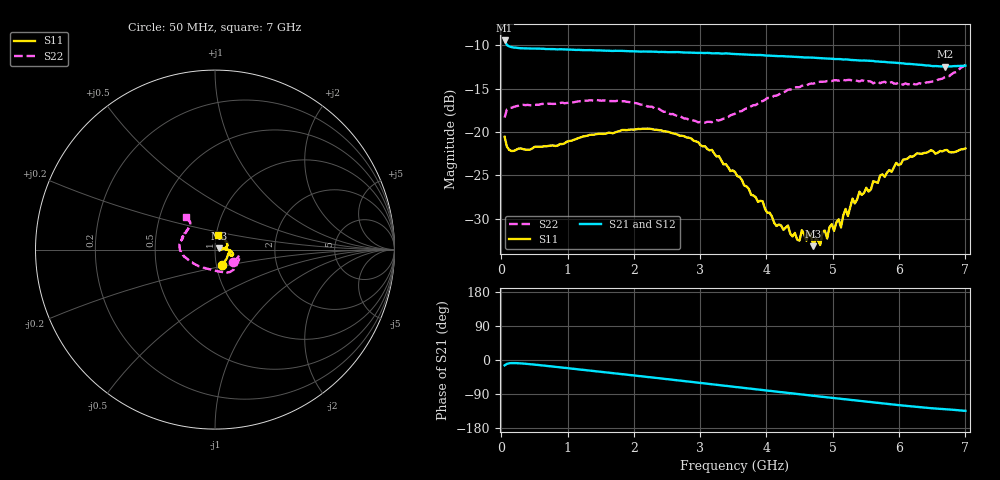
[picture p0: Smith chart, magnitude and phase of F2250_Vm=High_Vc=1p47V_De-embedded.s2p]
! Integrated Device Technology
! Corporate Headquarters
! 6024 Silver Creek Valley Road
! San Jose, CA 95138  USA
! Phone:  1-408-284-8200
! Toll Free:  1-800-223-1366
! Webpage:  http://www.idt.com/
! Timing and RF Division
! 515 Groton Road, Suite 102
! Westford, MA 01886-6024
! Device:  F2250
! Description: Voltage Variable RF Attenuator
! Frequency:  50.0 -  6000.00 MHz
! Package:  3x3 mm Thin QFN Plastic Package: 16 pin
! Ports:  2 RF, 3 DC
!  Pin  1  = GND
!  Pin  2  = NC
!  Pin  3  = RF1  = Port 1
!  Pin  4  = NC
!  Pin  5  = GND
!  Pin  6  = GND
!  Pin  7  = GND
!  Pin  8  = GND
!  Pin  9  = NC
!  Pin 10  = RF2  = Port 2
!  Pin 11  = NC
!  Pin 12  = GND
!  Pin 13  = GND
!  Pin 14  = VCNTRL
!  Pin 15  = VDD
!  Pin 16  = VMODE
! Vcntrl:  1.470 Volts
! Vmode:  +3.300 Volts
! Vdd:  +3.30  Volts
! Current:  1.331 mA
! Data:  The device was measured on a the F2250 evaluation board which has
!  individual transmission lines to the RF pins.  Data was collected
!  using a calibrated network analyzer.  The evaluation board was
!  de-embedded using a TRL calibration technique.
!  The reference plane is the edge of the package pin.
! Misc:  SN 10
!  Action Tracker AT0258
! Date Measured:  2014-11-26
! Date:  2015-10-15  MJV
! Note:
!  Integrated Device Technology supplies this data as a sample of measured
!  data at the package pin for this product.  Your particular data for this
!  product may vary.
!  Data was taken at 25 degrees C.
!  Integrated Device Technology reserves the right to change this data at anytime.
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# GHz S dB R 50
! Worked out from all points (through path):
!   201 points, 50 MHz to 7 GHz, reference 50 ohm
!   highest |S21| = -9.44 dB at 50 MHz (marker M1); lowest = -12.5 dB at 6.687 GHz (marker M2)
!   group delay of S21, straight-line fit = 53.4 ps
!   lowest |S11| = -33.2 dB at 4.707 GHz (marker M3), VSWR 1.04, Z = 52.1 + j0.658 ohm
!   |S11| at or under -10 dB: start of sweep to end of sweep
!   |S22| runs from -18.9 to -12.3 dB; largest |S21 - S12| = 0.0013
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0.05  -20.55 -64.2  -9.44 -14.3  -9.44 -14.3  -18.34 -34.1
0.15425  -22.20 -23.2  -10.20 -8.2  -10.20 -8.2  -17.20 -13.3
1.2315  -20.52 -20.1  -10.55 -25.9  -10.58 -25.9  -16.39 -42.0
2.37825  -19.80 -12.6  -10.77 -48.0  -10.78 -48.1  -17.33 -69.4
2.969  -21.17 -4.0  -10.87 -59.8  -10.86 -59.9  -18.88 -97.5
3.525  -24.62 2.6  -11.00 -71.0  -11.02 -71.0  -17.90 -132.9
4.1505  -30.86 12.0  -11.24 -83.4  -11.23 -83.5  -15.81 -160.9
4.32425  -30.81 13.0  -11.29 -86.9  -11.27 -87.0  -15.12 -166.6
4.498  -32.55 9.2  -11.35 -90.3  -11.36 -90.4  -14.84 -171.7
4.53275  -31.34 12.1  -11.37 -91.0  -11.38 -91.1  -14.67 -172.6
4.60225  -32.56 13.6  -11.40 -92.4  -11.38 -92.5  -14.63 -174.2
4.637  -31.57 12.4  -11.40 -93.2  -11.40 -93.2  -14.49 -175.3
4.7065  -33.19 16.7  -11.42 -94.5  -11.43 -94.5  -14.43 -176.3
4.81075  -33.06 9.2  -11.48 -96.5  -11.49 -96.5  -14.21 -178.4
4.8455  -31.47 6.7  -11.51 -97.2  -11.50 -97.2  -14.21 -179.2
4.915  -32.31 10.2  -11.52 -98.6  -11.52 -98.6  -14.13 178.8
5.08875  -30.09 11.1  -11.59 -102.0  -11.60 -102.0  -14.08 174.8
5.1235  -31.03 7.7  -11.60 -102.7  -11.60 -102.7  -14.02 173.8
5.29725  -27.69 6.7  -11.69 -105.9  -11.67 -106.0  -14.08 170.2
5.85325  -24.40 9.8  -11.96 -116.5  -11.96 -116.6  -14.36 155.0
6.68725  -22.11 45.2  -12.45 -129.7  -12.44 -129.9  -13.68 132.0
7  -21.90 78.3  -12.34 -134.2  -12.36 -134.3  -12.26 132.2
